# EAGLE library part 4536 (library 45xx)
Programmable TIMER
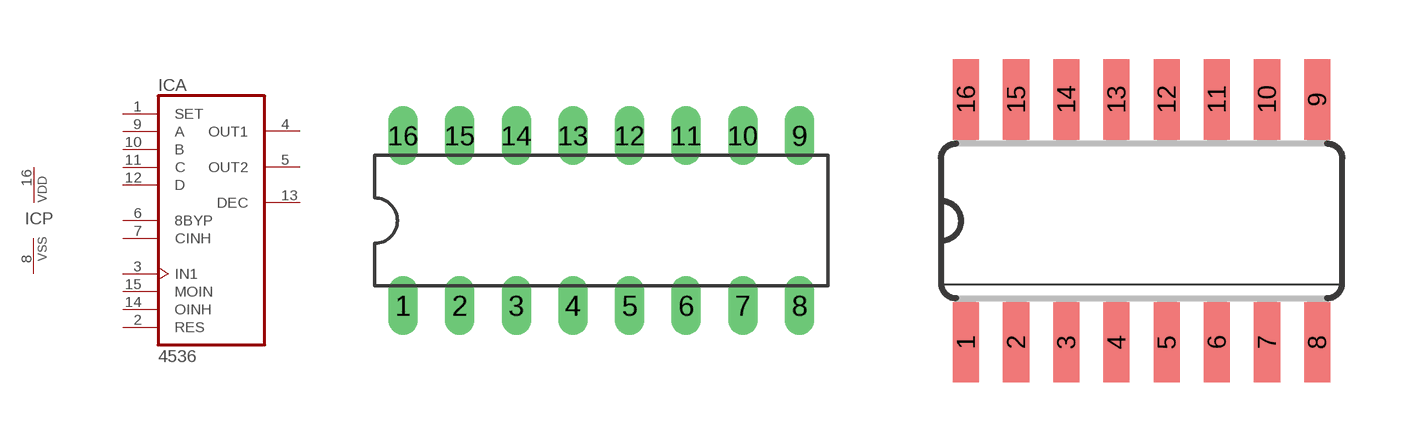
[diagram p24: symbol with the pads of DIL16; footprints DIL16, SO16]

Designator prefix IC; gates A=4536 P=PWRN

## 4536N  [DIL16]
1  A:SET  in
2  A:RES  in
3  A:IN1  in
4  A:OUT1  out
5  A:OUT2  out
6  A:8BYP  in
7  A:CINH  in
8  P:VSS  pwr
9  A:A  in
10  A:B  in
11  A:C  in
12  A:D  in
13  A:DEC  out
14  A:OINH  in
15  A:MOIN  in
16  P:VDD  pwr

## 4536D  [SO16]
Pads as for DIL16

## Footprint DIL16 (pad centres in mm)
Dual In Line Package
drill 0.813 long: 1 -8.89,-3.81; 2 -6.35,-3.81; 3 -3.81,-3.81; 4 -1.27,-3.81; 5 1.27,-3.81; 6 3.81,-3.81; 7 6.35,-3.81; 8 8.89,-3.81; 9 8.89,3.81; 10 6.35,3.81; 11 3.81,3.81; 12 1.27,3.81; 13 -1.27,3.81; 14 -3.81,3.81; 15 -6.35,3.81; 16 -8.89,3.81

## Footprint SO16 (pad centres in mm)
Small Outline package 150 mil
smd 0.66 x 2.032: 1 -4.445,-3.073; 2 -3.175,-3.073; 3 -1.905,-3.073; 4 -0.635,-3.073; 5 0.635,-3.073; 6 1.905,-3.073; 7 3.175,-3.073; 8 4.445,-3.073; 9 4.445,3.073; 10 3.175,3.073; 11 1.905,3.073; 12 0.635,3.073; 13 -0.635,3.073; 14 -1.905,3.073; 15 -3.175,3.073; 16 -4.445,3.073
